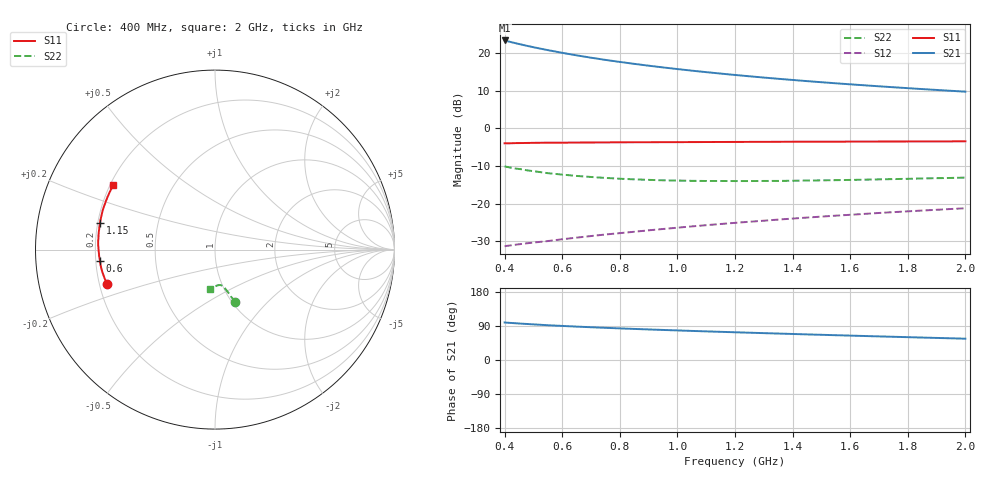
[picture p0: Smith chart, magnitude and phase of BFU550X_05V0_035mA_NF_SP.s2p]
! Filename:  P:\Prog\Test\Noise\ATS_data\Testdata_Net\BFU550X attenuator noise\BFU550X_APG2013_44_C05_05p0V_035mA_NF_CM01_D.sf
! Date/Time: Fri 26/Jul/2013 14:34:21
! BFU550X_APG2013_44_C05_05p0V_1to35mA_NF_CM01_Bias8_R.sf
! Noise Parameter Data File
! BFU550X_APG2013_44_C05_05p0V_1to35mA_NF_CM01
! Date/time: Mon Jul 22 09:12:23 2013
! VAR V_out= 5.001000
! VAR I_out= 34.995000
! VAR V_in= 0.821800
! VAR I_in= 0.395450
! Device data file deembeded for feedlines and parallel
! Original file: \BFU550X attenuator noise\BFU550X_APG2013_44_C05_05p0V_035mA_NF_CM01_R.sf
! Feed-files: PR005V01_100713_Feed1.s2p, PR005V01_100713_Feed2.s2p
! Parallel-file: PR005V01_100713_Par.s2p
# MHz S MA R 50
!  Freq-MHz  S11-mag  S11-arg  S21-mag  S21-arg  S12-mag  S12-arg  S22-mag  S22-arg
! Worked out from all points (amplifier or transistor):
!   37 points, 400 MHz to 2 GHz, reference 50 ohm
!   highest |S21| = 23.4 dB at 400 MHz (marker M1)
!   |S21| within 3 dB of that: start of sweep to 580 MHz
!   unconditionally stable (mu >= 1): 1.034 GHz to end of sweep
!   at 500 MHz: K = 0.78, MSG = 26.0 dB, |S12| = -30.4 dB
!   at 1.1 GHz: K = 1.01, MAG = 19.8 dB, |S12| = -25.8 dB
!   at 2 GHz: K = 1.06, MAG = 14.0 dB, |S12| = -21.3 dB
!   lowest NFmin = 1.33 dB at 480 MHz
!   S11 on the Smith chart (normalised r, x): 400 MHz: 0.23, -0.15; 600 MHz: 0.22, -0.05; 1.15 GHz: 0.21, +0.11; 2 GHz: 0.21, +0.28
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400  0.6321 -162.6  14.72 99.0  0.02709 50.4  0.3114 -68.8
420  0.6325 -164.0  14.07 97.9  0.02773 50.9  0.3005 -69.6
440  0.6356 -165.4  13.49 96.9  0.02838 51.3  0.2908 -69.9
480  0.6388 -168.0  12.43 94.9  0.02966 52.0  0.2752 -71.3
500  0.6408 -169.2  11.97 94.0  0.03025 52.4  0.2693 -71.6
550  0.6435 -172.2  10.95 91.8  0.03168 53.7  0.2531 -72.6
600  0.6436 -174.5  10.08 89.9  0.03349 54.7  0.2424 -73.7
650  0.6464 -176.7  9.33 88.1  0.0352 55.6  0.2326 -74.5
700  0.6475 -178.7  8.687 86.5  0.03692 56.5  0.2253 -75.3
750  0.6495 179.4  8.121 84.9  0.03872 57.2  0.2189 -76.2
800  0.6516 177.6  7.631 83.4  0.04038 57.9  0.2135 -77.2
850  0.6527 175.8  7.192 82.0  0.0421 58.7  0.2094 -78.0
900  0.6527 174.2  6.797 80.6  0.04399 59.3  0.2062 -78.8
950  0.6543 172.7  6.45 79.3  0.04584 59.8  0.2035 -79.5
1050  0.6555 169.8  5.842 76.8  0.04961 60.7  0.2002 -81.2
1150  0.6579 167.1  5.34 74.3  0.05342 61.3  0.1993 -82.8
1200  0.6588 165.7  5.12 73.2  0.05532 61.5  0.1988 -83.6
1350  0.6617 161.9  4.553 69.8  0.06112 62.1  0.1997 -86.1
1500  0.664 158.3  4.1 66.5  0.06694 62.3  0.2032 -88.7
1600  0.6651 156.0  3.844 64.4  0.07079 62.4  0.2059 -90.2
1750  0.6671 152.7  3.515 61.3  0.07678 62.3  0.2112 -92.8
2000  0.6714 147.5  3.071 56.2  0.08649 61.9  0.2212 -96.9
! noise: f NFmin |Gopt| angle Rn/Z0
400  1.422  0.3818  -172.4  0.0791
460  1.333  0.4151  -169.9  0.0721
600  1.346  0.4262  -169  0.0696
800  1.35  0.4415  -166.1  0.0707
1000  1.37  0.4843  -162.3  0.0626
1200  1.438  0.4913  -159  0.0682
1400  1.468  0.4907  -154.9  0.0786
1600  1.507  0.511  -149.2  0.0896
1800  1.545  0.4893  -148.9  0.0994
2000  1.618  0.5175  -143.6  0.1128
